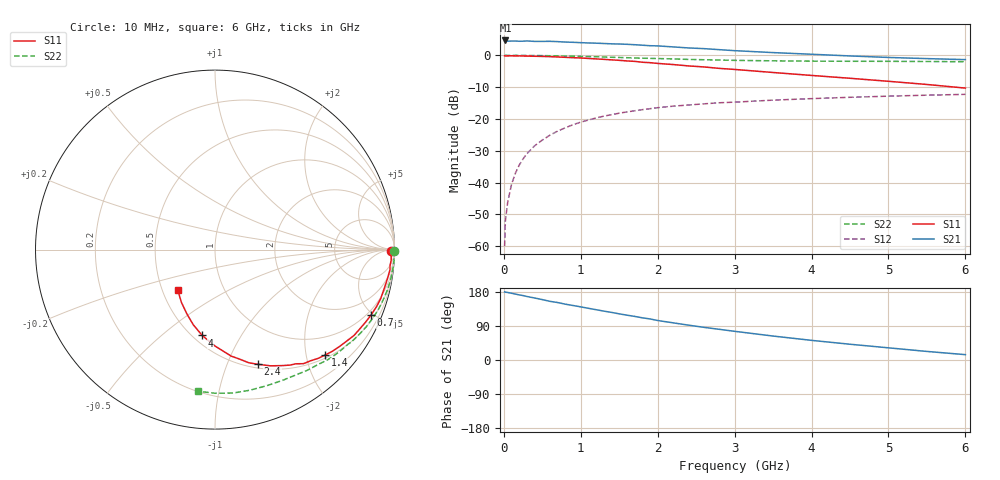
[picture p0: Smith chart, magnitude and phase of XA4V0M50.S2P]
! SIEMENS Discrete & RF Semiconductors
! BFY180
! Si NPN RF Bipolar Junction Transistor in MICRO-X
! VCE = 4 V  IC = 0.5 mA
! Common Emitter S-Parameters:  May  1997
# GHz  S  MA  R  50
!  f  S11  S21  S12  S22
! GHz  MAG  ANG  MAG  ANG  MAG  ANG  MAG  ANG
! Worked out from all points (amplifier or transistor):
!   36 points, 10 MHz to 6 GHz, reference 50 ohm
!   highest |S21| = 4.7 dB at 20 MHz (marker M1)
!   |S21| within 3 dB of that: start of sweep to 2.867 GHz
!   unconditionally stable (mu >= 1): 5.738 GHz to end of sweep
!   at 250 MHz: K = 0.06, MSG = 18.5 dB, |S12| = -32.5 dB
!   at 1.4 GHz: K = 0.39, MSG = 11.1 dB, |S12| = -18.7 dB
!   at 6 GHz: K = 1.01, MAG = 4.9 dB, |S12| = -12.3 dB
!   S11 on the Smith chart (normalised r, x): 10 MHz: open; 700 MHz: 0.74, -4.85; 1.4 GHz: 0.56, -2.37; 2.4 GHz: 0.54, -1.29; 4 GHz: 0.56, -0.69; 6 GHz: 0.60, -0.30
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0.01  0.9829 -0.4  1.676 179.7  0.001 85.4  0.9988 -0.3
0.02  0.9771 -0.5  1.715 179.1  0.0025 87.5  0.9999 -0.5
0.05  0.9813 -1.6  1.672 178.2  0.0049 85.5  0.9985 -1.1
0.1  0.9839 -3.3  1.678 176.1  0.0094 88.4  0.9962 -2.3
0.15  0.9793 -5.2  1.679 174.0  0.014 86.4  0.9993 -3.4
0.2  0.9814 -6.5  1.666 171.8  0.0188 85.9  0.9979 -4.5
0.3  0.9737 -9.8  1.686 167.6  0.0285 82.0  0.9953 -6.8
0.4  0.9678 -12.8  1.657 163.6  0.0378 80.2  0.9936 -9.0
0.6  0.9546 -19.4  1.662 154.8  0.0557 74.9  0.986 -13.4
0.7  0.9426 -22.8  1.644 151.6  0.0645 72.1  0.9804 -15.6
1.1  0.8939 -34.7  1.566 136.4  0.0961 62.8  0.9562 -24.0
1.4  0.8495 -43.8  1.518 125.6  0.1168 55.8  0.9332 -30.2
1.7  0.8043 -52.2  1.471 115.1  0.1344 50.2  0.9082 -35.7
2  0.7471 -59.9  1.408 104.2  0.1504 44.8  0.8911 -40.8
2.2  0.7174 -64.5  1.358 98.1  0.1589 41.2  0.8782 -44.3
2.4  0.6822 -69.5  1.308 92.0  0.1658 38.2  0.8633 -47.3
3  0.6007 -81.3  1.185 75.7  0.1838 30.0  0.8344 -56.0
3.5  0.5378 -89.9  1.105 63.2  0.1977 24.6  0.8201 -62.6
4  0.4834 -98.5  1.041 51.8  0.2088 19.4  0.8112 -69.2
4.5  0.4361 -106.1  0.979 41.6  0.2191 14.5  0.8072 -76.0
5.5  0.3485 -122.5  0.889 22.6  0.2365 5.5  0.8004 -89.9
6  0.3057 -132.8  0.857 14.1  0.2437 0.7  0.795 -96.9
